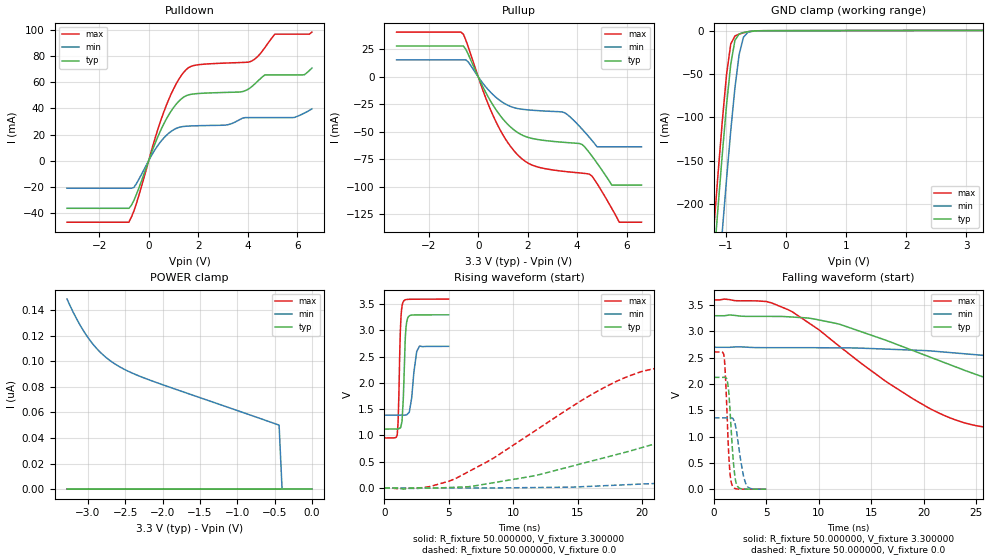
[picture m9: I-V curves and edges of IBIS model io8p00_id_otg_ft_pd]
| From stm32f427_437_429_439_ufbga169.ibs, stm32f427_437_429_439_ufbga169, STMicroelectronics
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|   Model io8p00_id_otg_ft_pd
[Model]  io8p00_id_otg_ft_pd
Model_type I/O
Polarity   Non-Inverting
Enable   Active-Low
Vinl =   0.990000V
Vinh =   2.310000V
Vmeas =  1.650000V
Cref =   50.000000pF
Rref =   100.000000M
Vref =   0.0V
C_comp   2.282200pF   2.214200pF   2.357400pF
[Temperature Range]   25.000000   0.125000k   -40.000000
[Pullup Reference]   3.300000V   2.700000V   3.600000V
[Pulldown Reference]   0.0V   0.0V   0.0V
[POWER Clamp Reference]   3.300000V   2.700000V   3.600000V
[GND Clamp Reference]   0.0V   0.0V   0.0V
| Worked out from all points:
|   slope of the pulldown table from 0 to 0.495 V, typ, clamps not added: 20.9 ohm
|   slope of the pullup table from 0 to 0.495 V, typ, clamps not added: 22.6 ohm
|   GND clamp passes 1 mA (typ) near -0.62 V on its own axis
|   rising waveform, R_fixture 50.000000, V_fixture 3.300000: 20-80 % time 190ps typ, 342ps min, 164ps max; typ from 1.12 V to 3.29 V
|   rising waveform, R_fixture 50.000000, V_fixture 0.0: 20-80 % time 19.8ns typ, 51.1ns min, 10.4ns max; typ from 0 V to 2.12 V
|   falling waveform, R_fixture 50.000000, V_fixture 3.300000: 20-80 % time 18.9ns typ, 39.6ns min, 11.4ns max; typ from 3.29 V to 1.12 V
|   falling waveform, R_fixture 50.000000, V_fixture 0.0: 20-80 % time 432ps typ, 632ps min, 342ps max; typ from 2.12 V to 0 V
[Pulldown]
|Voltage   I(typ)   I(min)   I(max)
-3.3V     -36.46mA   -21.1mA    -47.09mA
-800mV    -36.46mA   -21.1mA    -47.09mA
-600mV    -30.5mA    -20.54mA   -38.68mA
700mV     31.39mA    19.1mA     41.7mA
1.2V      45.14mA    25.37mA    61.74mA
1.6V      50.34mA    26.49mA    71.04mA
3.1V      52.26mA    27.25mA    74.74mA
4.1V      55.69mA    32.98mA    75.78mA
4.7V      65.7mA     32.98mA    86.67mA
5.1V      65.7mA     32.98mA    96.88mA
6.3V      65.85mA    36.49mA    96.88mA
6.6V      70.9mA     39.7mA     98.46mA
[Pullup]
|Voltage   I(typ)   I(min)   I(max)
-3.3V     28.03mA    15.42mA    40.69mA
-700mV    28.03mA    15.42mA    40.69mA
-400mV    20.31mA    13.47mA    26.93mA
600mV     -25.77mA   -16.23mA   -35.13mA
1.6V      -50.64mA   -28.8mA    -70.96mA
3.5V      -59.53mA   -32.65mA   -85.92mA
4.2V      -61.43mA   -47.48mA   -87.46mA
4.5V      -69.07mA   -55.13mA   -88.38mA
4.8V      -78.22mA   -63.5mA    -96.83mA
5.4V      -98.3mA    -63.5mA    -119.6mA
5.7V      -98.3mA    -63.5mA    -132mA
6.6V      -98.3mA    -63.5mA    -132mA
[GND_clamp]
|Voltage   I(typ)   I(min)   I(max)
-3.3V     -2.318A    -2.397A    -2.291A
-1.2V     -265.5mA   -356.1mA   -227.2mA
-1.13V    -202.7mA   -292.9mA   -164.2mA
-1.06V    -142.2mA   -231.2mA   -104.1mA
-990mV    -86mA      -171.6mA   -50.76mA
-920mV    -38.84mA   -115.5mA   -15.35mA
-850mV    -11.15mA   -65.63mA   -6.09mA
-780mV    -3.853mA   -27.45mA   -3.961mA
-710mV    -2.153mA   -7.739mA   -2.46mA
-640mV    -1.209mA   -2.169mA   -1.292mA
-570mV    -580.3uA   -846.3uA   -542.8uA
3.28V     342.5uA    239.2uA    398.5uA
[POWER_clamp]
|Voltage   I(typ)   I(min)   I(max)
-3.28V    0A         148.5nA    0A
-3.2V     0A         138.6nA    0A
-3.12V    0A         129.7nA    0A
-3.04V    0A         122nA      0A
-2.96V    0A         115.3nA    0A
-2.8V     0A         105.1nA    0A
-2.6V     0A         96.44nA    0A
-2.4V     0A         90.52nA    0A
-2.16V    0A         84.97nA    0A
-440mV    0A         50.04nA    0A
-400mV    0A         0A         0A
0V        0A         0A         0A
[Ramp]
| variable   typ   min   max
dV/dt_r  1.27434/19.74955n   0.81270/51.08570n   1.56402/10.36122n
dV/dt_f  1.30590/18.87704n   0.78546/39.67385n   1.58593/11.36713n
R_load = 50.000000
[Rising Waveform]
R_fixture= 50.000000
V_fixture= 3.300000
V_fixture_min= 2.700000
V_fixture_max= 3.600000
|time   V(typ)   V(min)   V(max)
0s        1.121V     1.386V     951.7mV
1.001ns   1.123V     1.387V     1.016V
1.071ns   1.125V     1.387V     1.287V
1.251ns   1.146V     1.387V     3.035V
1.461ns   1.657V     1.385V     3.541V
1.632ns   2.881V     1.388V     3.582V
1.862ns   3.257V     1.425V     3.59V
2.503ns   3.294V     2.584V     3.592V
2.723ns   3.294V     2.698V     3.593V
4.985ns   3.295V     2.695V     3.595V
[Rising Waveform]
R_fixture= 50.000000
V_fixture= 0.0
V_fixture_min= 0.0
V_fixture_max= 0.0
|time   V(typ)   V(min)   V(max)
0s        4.824nV    241.4nV    3.053nV
5.506ns   13.76mV    -139.7uV   177mV
11.51ns   226.5mV    8.227mV    1.059V
19.02ns   700.7mV    64.61mV    2.134V
27.53ns   1.282V     162.7mV    2.482V
38.04ns   1.834V     349.9mV    2.57V
55.06ns   2.051V     660.3mV    2.603V
89.59ns   2.113V     1.14V      2.607V
118.1ns   2.123V     1.295V     2.607V
249.2ns   2.124V     1.354V     2.607V
[Falling Waveform]
R_fixture= 50.000000
V_fixture= 3.300000
V_fixture_min= 2.700000
V_fixture_max= 3.600000
|time   V(typ)   V(min)   V(max)
0s        3.295V     2.695V     3.595V
5.506ns   3.282V     2.688V     3.538V
12.01ns   3.132V     2.684V     2.708V
22.02ns   2.402V     2.604V     1.396V
30.53ns   1.789V     2.446V     1.083V
36.04ns   1.497V     2.314V     1.037V
45.55ns   1.282V     2.082V     998.6mV
62.56ns   1.183V     1.732V     968.5mV
89.59ns   1.139V     1.508V     954.9mV
249.2ns   1.121V     1.386V     951.7mV
[Falling Waveform]
R_fixture= 50.000000
V_fixture= 0.0
V_fixture_min= 0.0
V_fixture_max= 0.0
|time   V(typ)   V(min)   V(max)
0s        2.124V     1.354V     2.607V
981ps     2.125V     1.354V     2.501V
1.151ns   2.115V     1.354V     1.938V
1.411ns   1.864V     1.355V     677.1mV
1.542ns   1.482V     1.356V     291.1mV
1.742ns   826.4mV    1.349V     73.99mV
2.152ns   97.4mV     1.115V     6.399mV
2.573ns   9.304mV    522.6mV    886.5uV
3.123ns   833.7uV    71.25mV    75.93uV
4.985ns   4.824nV    241.4nV    3.053nV
